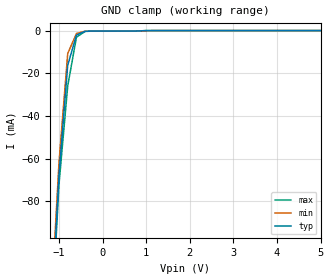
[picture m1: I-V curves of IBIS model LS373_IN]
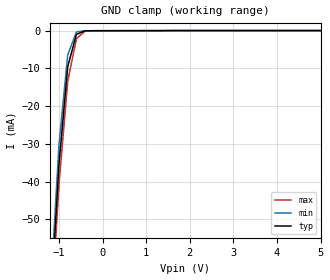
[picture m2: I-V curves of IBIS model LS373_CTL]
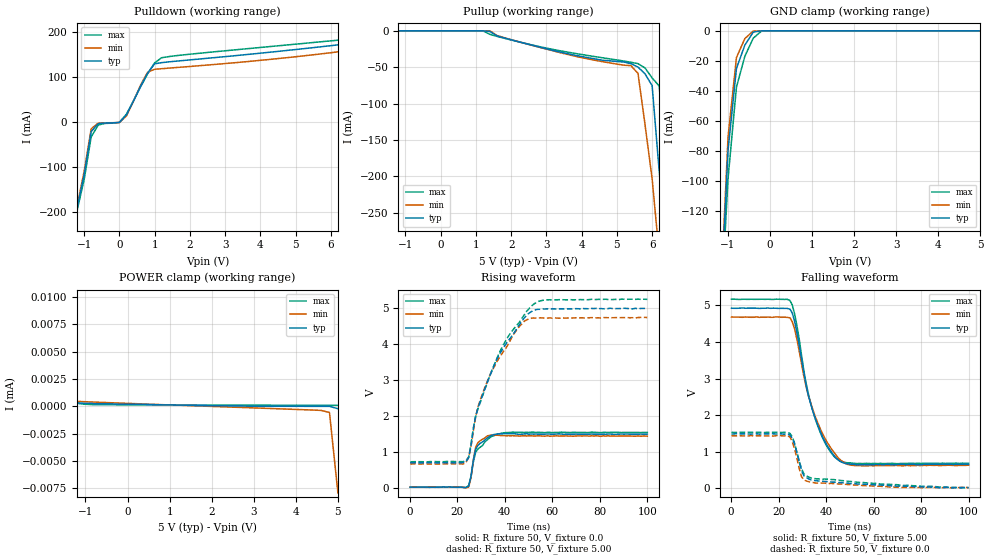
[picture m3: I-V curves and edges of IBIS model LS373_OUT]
|   TEXAS INSTRUMENTS INCORPORATED
|   Standard Linear and Logic Group
|   IBIS Model of SN74LS373
|   OCTAL D-TYPE TRANSPARENT LATCHES AND EDGE TRIGGERED FLIP-FLOPS
|   PDIP 20-pin(N), SOP 20-pin(NS), SOIC 20-pin(DW)
[IBIS Ver]   3.1
[Comment Char]  |_char
[File Name]   sn74ls373.ibs
[File Rev]   1.1
[Date]   July 13, 2004
[Source]   File originated at Texas Instruments, Inc.
[Notes]   - All test data contained in this file are derived from
   actual measurements.
   - FILE REV HISTORY
   - 1.1 Release IBIS file on 07/15/04
   - The measurement used NS package.
[Disclaimer] Property of Texas Instruments Incorporated.  Unauthorized
   reproduction and/or distribution is strictly prohibited.
   This product is protected under copyright law.
   Created 2000, (C) Copyright 2000, Texas Instruments Inc.,
   All Rights Reserved.
   UNLESS THERE IS A SIGNED, WRITTEN AGREEMENT TO THE
   CONTRARY, TEXAS INSTRUMENTS () IS PROVIDING THE IBIS
   MODELS  AND WITHOUT ANY WARRANTY, EXPRESSED OR
   IMPLIED.  TI assumes no liability for:
   1) the accuracy of the IBIS models provided to your
   company;
   2) the proper functioning of these IBIS Models in your
   design or for any resulting applications; or
   3) infringement of patents, copyrights or intellectual
   property rights resulting from your use of these IBIS
   models.
   TI provides IBIS Models as a service to our customers.
   You and your company shall not distribute, sell or give
   these models to anyone else without prior written
   permission from TI.
   TI reserves the right to make changes to our products or
   to discontinue any semiconductor product or service
   without notice, and advises our customers to obtain the
   latest version of relevant information to verify, before
   placing orders, that the information being relied on is
   current.
   Please be aware that your receipt and use of the IBIS
   information provided shall serve as acceptance of these
   terms and conditions.  If you do not accept these terms,
   you should return or destroy the IBIS models and any
   other accompanying information immediately.
|   Component LS373_N
[Component]   LS373_N
[Manufacturer]  Texas Instruments, Inc.
[Package]
|   typ   min   max
R_pkg   0.038   0.033   0.045
L_pkg   5.012nH   4.110nH   6.349nH
C_pkg   0.717pF   0.530pF   0.868pF
[Pin]   signal_name   model_name   R_pin   L_pin   C_pin
1   OC_NOT   LS373_CTL   0.058   5.115nH   0.725pF
2   1Q   LS373_OUT   0.053   4.591nH   0.724pF
3   1D   LS373_IN   0.049   3.754nH   0.572pF
4   2D   LS373_IN   0.029   2.549nH   0.388pF
5   2Q   LS373_OUT   0.031   2.317nH   0.316pF
6   3Q   LS373_OUT   0.031   2.317nH   0.316pF
7   3D   LS373_IN   0.029   2.556nH   0.399pF
8   4D   LS373_IN   0.049   3.754nH   0.579pF
9   4Q   LS373_OUT   0.053   4.591nH   0.724pF
10   GND   GND   0.058   5.115nH   0.725pF
11   C   LS373_IN   0.058   5.115nH   0.725pF
12   5Q   LS373_OUT   0.053   4.591nH   0.724pF
13   5D   LS373_IN   0.049   3.754nH   0.579pF
14   6D   LS373_IN   0.029   2.557nH   0.399pF
15   6Q   LS373_OUT   0.031   2.317nH   0.316pF
16   7Q   LS373_OUT   0.031   2.317nH   0.316pF
17   7D   LS373_IN   0.029   2.557nH   0.399pF
18   8D   LS373_IN   0.049   3.754nH   0.579pF
19   8Q   LS373_OUT   0.053   4.591nH   0.724pF
20   VCC   POWER   0.058   5.115nH   0.725pF
|   Component LS373_NS
[Component]   LS373_NS
[Manufacturer]  Texas Instruments, Inc.
[Package]
|   typ   min   max
R_pkg   0.044   0.029   0.058
L_pkg   3.666nH   2.317nH   5.115nH
C_pkg   0.548pF   0.316pF   0.725pF
[Pin]   signal_name   model_name   R_pin   L_pin   C_pin
1   OC_NOT   LS373_CTL   0.058   5.115nH   0.725pF
2   1Q   LS373_OUT   0.053   4.591nH   0.724pF
3   1D   LS373_IN   0.049   3.754nH   0.572pF
4   2D   LS373_IN   0.029   2.549nH   0.388pF
5   2Q   LS373_OUT   0.031   2.317nH   0.316pF
6   3Q   LS373_OUT   0.031   2.317nH   0.316pF
7   3D   LS373_IN   0.029   2.556nH   0.399pF
8   4D   LS373_IN   0.049   3.754nH   0.579pF
9   4Q   LS373_OUT   0.053   4.591nH   0.724pF
10   GND   GND   0.058   5.115nH   0.725pF
11   C   LS373_IN   0.058   5.115nH   0.725pF
12   5Q   LS373_OUT   0.053   4.591nH   0.724pF
13   5D   LS373_IN   0.049   3.754nH   0.579pF
14   6D   LS373_IN   0.029   2.557nH   0.399pF
15   6Q   LS373_OUT   0.031   2.317nH   0.316pF
16   7Q   LS373_OUT   0.031   2.317nH   0.316pF
17   7D   LS373_IN   0.029   2.557nH   0.399pF
18   8D   LS373_IN   0.049   3.754nH   0.579pF
19   8Q   LS373_OUT   0.053   4.591nH   0.724pF
20   VCC   POWER   0.058   5.115nH   0.725pF
|   ComponentLS373_DW
[Component]   LS373_DW
[Manufacturer]  Texas Instruments, Inc.
[Package]
|   typ   min   max
R_pkg   0.038   0.033   0.045
L_pkg   5.012nH   4.110nH   6.349nH
C_pkg   0.717pF   0.530pF   0.868pF
[Pin]   signal_name   model_name   R_pin   L_pin   C_pin
1   OC_NOT   LS373_CTL   0.058   5.115nH   0.725pF
2   1Q   LS373_OUT   0.053   4.591nH   0.724pF
3   1D   LS373_IN   0.049   3.754nH   0.572pF
4   2D   LS373_IN   0.029   2.549nH   0.388pF
5   2Q   LS373_OUT   0.031   2.317nH   0.316pF
6   3Q   LS373_OUT   0.031   2.317nH   0.316pF
7   3D   LS373_IN   0.029   2.556nH   0.399pF
8   4D   LS373_IN   0.049   3.754nH   0.579pF
9   4Q   LS373_OUT   0.053   4.591nH   0.724pF
10   GND   GND   0.058   5.115nH   0.725pF
11   C   LS373_IN   0.058   5.115nH   0.725pF
12   5Q   LS373_OUT   0.053   4.591nH   0.724pF
13   5D   LS373_IN   0.049   3.754nH   0.579pF
14   6D   LS373_IN   0.029   2.557nH   0.399pF
15   6Q   LS373_OUT   0.031   2.317nH   0.316pF
16   7Q   LS373_OUT   0.031   2.317nH   0.316pF
17   7D   LS373_IN   0.029   2.557nH   0.399pF
18   8D   LS373_IN   0.049   3.754nH   0.579pF
19   8Q   LS373_OUT   0.053   4.591nH   0.724pF
20   VCC   POWER   0.058   5.115nH   0.725pF
| Models and submodels in the file (3): LS373_IN (Input), LS373_CTL (Input), LS373_OUT (Output)
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|   Model LS373_IN
[Model]   LS373_IN
Model_type  Input
Polarity   Non-Inverting
Vinl = 0.8
Vinh = 2.0
| variable   typ   min   max
C_comp   1.33pf   1.00pf   1.66pf
[Temperature Range]   25   0   70
[Voltage Range]   5.00   4.75   5.25
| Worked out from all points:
|   GND clamp passes 1 mA (typ) near -0.48 V on its own axis
[GND Clamp]
|   Voltage   I(typ)   I(min)   I(max)
-5V       -2.128A    -2.306A    -2.005A
-1.2V     -143.6mA   -135.9mA   -148.2mA
-1V       -67.59mA   -61.94mA   -72.12mA
-800mV    -16.28mA   -10.76mA   -26mA
-600mV    -2.116mA   -1.383mA   -3.124mA
-400mV    -303uA     -281.8uA   -391.1uA
-200mV    -246.9uA   -263.1uA   -237.3uA
5V        225.4pA    365.5nA    759.5pA
|   Model LS373_CTL
[Model]   LS373_CTL
Model_type  Input
Polarity   Inverting
Vinl = 0.8
Vinh = 2.0
| variable   typ   min   max
C_comp   1.35pf   1.01pf   1.69pf
[Temperature Range]   25   0   70
[Voltage Range]   5.00   4.75   5.25
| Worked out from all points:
|   GND clamp passes 1 mA (typ) near -0.60 V on its own axis
[GND Clamp]
|   Voltage   I(typ)   I(min)   I(max)
-5V       -1.031A    -1.09A     -965.2mA
-1.2V     -74.85mA   -70.27mA   -78.96mA
-1V       -35.35mA   -30.13mA   -40.75mA
-800mV    -9.565mA   -6.463mA   -13.44mA
-600mV    -1.001mA   -355.1uA   -2.17mA
-400mV    -49.37uA   -47.27uA   -104.2uA
5V        2.076nA    171.2nA    464.8pA
|   Model LS373_OUT
[Model]   LS373_OUT
Model_type  Output
Polarity   Non-Inverting
Vmeas = 1.3v
Cref = 45pf
Rref = 667
Vref = 0
| variable   typ   min   max
C_comp   5.80pf   4.35pf   7.25pf
[Temperature Range]   25   0   70
[Voltage Range]   5.00   4.75   5.25
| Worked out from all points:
|   slope of the pulldown table from 0 to 0.75 V, typ, clamps not added: 7.33 ohm
|   GND clamp passes 1 mA (typ) near -0.40 V on its own axis
|   rising waveform, R_fixture 50, V_fixture 0.0: 20-80 % time 3.27ns typ, 2.13ns min, 5.37ns max; typ from 0.024 V to 1.5 V
|   falling waveform, R_fixture 50, V_fixture 5.00: 20-80 % time 9.61ns typ, 10.6ns min, 9.04ns max; typ from 4.92 V to 0.66 V
|   rising waveform, R_fixture 50, V_fixture 5.00: 20-80 % time 15.4ns typ, 14.3ns min, 16.1ns max; typ from 0.7 V to 4.99 V
|   falling waveform, R_fixture 50, V_fixture 0.0: 20-80 % time 4.45ns typ, 3.47ns min, 5.58ns max; typ from 1.49 V to 0.023 V
[Pulldown]
|   Voltage   I(typ)   I(min)   I(max)
-5V       -1.978A    -2.082A    -1.836A
-1.4V     -282.6mA   -282.4mA   -282.8mA
-1.2V     -192mA     -187.7mA   -197.7mA
-1V       -118.5mA   -110.9mA   -129.2mA
-800mV    -22.27mA   -15.99mA   -34.17mA
-600mV    -4.43mA    -3.35mA    -7.571mA
0V        -1.935mA   -2.026mA   -1.773mA
200mV     14.62mA    12.29mA    16.48mA
800mV     107.8mA    109.7mA    106mA
1.2V      131.1mA    117.6mA    142mA
6V        168.8mA    153.1mA    179.5mA
10V       203.9mA    199.5mA    209.6mA
[Pullup]
|   Voltage   I(typ)   I(min)   I(max)
-5V       9.772uA    5.735uA    29.06uA
1.2V      7.593uA    4.552uA    -52.29uA
1.4V      -925.2uA   -51uA      -4.883mA
3.4V      -29.32mA   -30.05mA   -27.49mA
5.4V      -45.11mA   -47.86mA   -43.17mA
5.6V      -49.81mA   -58.55mA   -45.11mA
5.8V      -59.22mA   -129.3mA   -51.08mA
6V        -75.25mA   -203.2mA   -64.7mA
6.2V      -192.3mA   -306.8mA   -75.8mA
6.4V      -282.7mA   -404.3mA   -179.9mA
6.6V      -374.5mA   -503.4mA   -262.3mA
10V       -1.973A    -2.198A    -1.715A
[GND Clamp]
|   Voltage   I(typ)   I(min)   I(max)
-5V       -1.963A    -2.071A    -1.826A
-1.2V     -196.6mA   -192mA     -202.4mA
-1V       -79.6mA    -70.73mA   -98.28mA
-800mV    -25.01mA   -17.77mA   -37.42mA
-600mV    -9.515mA   -5.14mA    -16.9mA
-400mV    -804.9uA   -175.2uA   -4.862mA
-200mV    -8.76uA    -3.296uA   -76.84uA
5V        186.2nA    178.7nA    213.7nA
[POWER Clamp]
|   Voltage   I(typ)   I(min)   I(max)
-5V       239.9uA    250.7uA    215.3uA
-1.6V     23.86uA    14.32uA    30.28uA
-1.4V     8.95uA     3.503uA    19.08uA
-1.2V     325.7nA    466.8nA    283.5nA
-800mV    265.6nA    399nA      163nA
2.4V      50.8nA     -51.05nA   121.3nA
4.6V      11.5nA     -361.2nA   108.7nA
4.8V      10.1nA     -550.8nA   108.4nA
5V        -205.7nA   -7.896uA   108.4nA
[Ramp]
| variable   typ   min   max
dV/dt_r   9.100E-01/3.380E-09   8.500E-01/2.150E-09   9.500E-01/5.120E-09
dV/dt_f   2.620E+00/9.800E-09   2.480E+00/1.087E-08   2.750E+00/9.310E-09
R_load = 50
[Rising Waveform]
R_fixture = 50
V_fixture = 0.0
V_fixture_min = 0.0
V_fixture_max = 0.0
C_fixture = 0pf
L_fixture = 0nH
|   Time   V(typ)   V(min)   V(max)
195.3ps   23.76mV    24.75mV    20.64mV
23.63ns   10.64mV    3.69mV     12.55mV
24.8ns    50.46mV    24.75mV    68.4mV
25.78ns   323.3mV    283.4mV    306.1mV
26.76ns   767.2mV    771.7mV    716.5mV
27.73ns   1.078V     1.127V     990.8mV
28.71ns   1.183V     1.26V      1.083V
33.59ns   1.429V     1.462V     1.393V
43.36ns   1.509V     1.454V     1.551V
100ns     1.498V     1.441V     1.542V
[Falling Waveform]
R_fixture = 50
V_fixture = 5.00
V_fixture_min = 4.75
V_fixture_max = 5.25
C_fixture = 0pf
L_fixture = 0nH
|   Time   V(typ)   V(min)   V(max)
195.3ps   4.924V     4.683V     5.171V
24.8ns    4.896V     4.661V     5.135V
26.76ns   4.57V      4.362V     4.771V
31.64ns   2.802V     2.774V     2.867V
34.57ns   2.085V     2.128V     2.09V
39.45ns   1.296V     1.378V     1.259V
45.31ns   767.8mV    823.2mV    773.2mV
49.22ns   675.1mV    652.3mV    700.5mV
53.13ns   643.9mV    622.3mV    678.1mV
100ns     660.1mV    636.3mV    688.8mV
[Rising Waveform]
R_fixture = 50
V_fixture = 5.00
V_fixture_min = 4.75
V_fixture_max = 5.25
C_fixture = 0pf
L_fixture = 0nH
|   Time   V(typ)   V(min)   V(max)
195.3ps   700.1mV    666.2mV    727.2mV
23.63ns   725.4mV    705.3mV    761.4mV
24.8ns    841.2mV    851mV      862.9mV
26.76ns   1.637V     1.572V     1.66V
28.71ns   2.224V     2.251V     2.202V
33.59ns   3.106V     3.111V     3.099V
39.45ns   3.897V     3.795V     3.982V
45.31ns   4.454V     4.421V     4.541V
52.15ns   4.934V     4.722V     5.106V
100ns     4.989V     4.737V     5.24V
[Falling Waveform]
R_fixture = 50
V_fixture = 0.0
V_fixture_min = 0.0
V_fixture_max = 0.0
C_fixture = 0pf
L_fixture = 0nH
|   Time   V(typ)   V(min)   V(max)
195.3ps   1.486V     1.44V      1.533V
20.12ns   1.492V     1.446V     1.53V
24.8ns    1.457V     1.407V     1.505V
25.78ns   1.37V      1.281V     1.41V
26.76ns   1.21V      1.077V     1.237V
29.69ns   488.3mV    319mV      536.1mV
30.66ns   348.5mV    238.8mV    400.4mV
33.59ns   234.8mV    169.1mV    290.3mV
69.73ns   62.38mV    33.3mV     104mV
100ns     23.47mV    22.62mV    19.27mV
